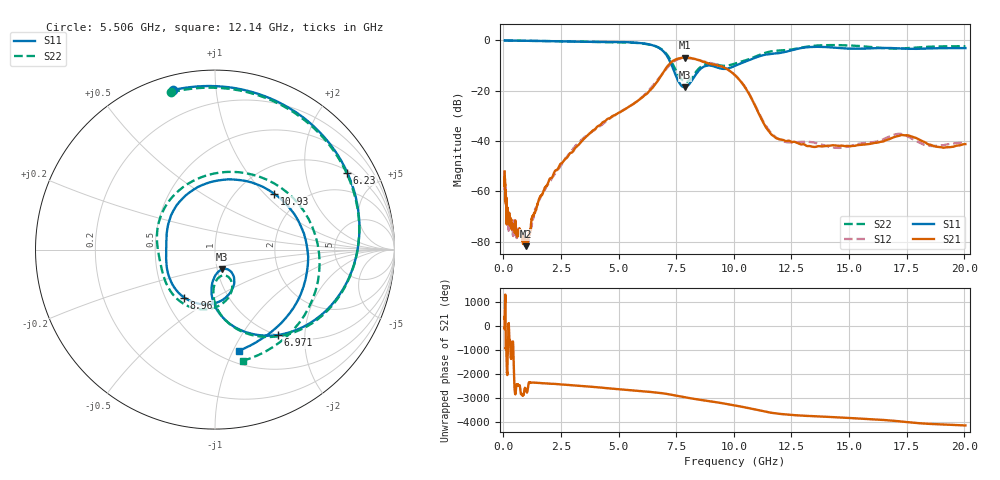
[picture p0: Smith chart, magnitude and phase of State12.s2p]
# Hz S DB R 50
!freq MagS11 AngS11 MagS21 AngS21 MagS12 AngS12 MagS22 AngS22
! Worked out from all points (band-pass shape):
!   1601 points, 50 MHz to 20.05 GHz, reference 50 ohm
!   highest |S21| = -6.81 dB at 7.859 GHz (marker M1); lowest = -81.9 dB at 964.4 MHz (marker M2)
!   |S21| within 3 dB of the highest: 7.16 GHz to 9.241 GHz (2.081 GHz wide, 25.4 % of centre)
!   lowest |S11| = -18.6 dB at 7.859 GHz (marker M3), VSWR 1.27, Z = 52.9 - j11.8 ohm
!   |S11| at or under -10 dB: 7.308 GHz to 8.859 GHz (1.551 GHz wide, 19.2 % of centre); 9.001 GHz to 10.07 GHz (1.069 GHz wide, 11.2 % of centre)
!   |S22| runs from -16.5 to 0.0 dB; largest |S21 - S12| = 0.024
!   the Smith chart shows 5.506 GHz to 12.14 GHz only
!   S11 on the Smith chart (normalised r, x): 5.506 GHz: 0.07, +0.77; 6.23 GHz: 1.08, +3.39; 6.971 GHz: 1.00, -1.46; 8.96 GHz: 0.62, -0.37; 10.93 GHz: 1.46, +1.14; 12.14 GHz: 0.62, -1.06
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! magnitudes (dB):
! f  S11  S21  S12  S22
! 50 MHz  0.0  -52.1  -51.8  0.0
! 72.18 MHz  0.0  -63.6  -60.0  0.0
! 135.9 MHz  0.0  -67.1  -65.3  0.0
! 144.3 MHz  0.0  -72.7  -66.7  0.0
! 174.7 MHz  0.0  -67.4  -71.3  0.0
! 208.4 MHz  0.0  -71.2  -69.6  0.0
! 226.3 MHz  0.0  -71.9  -75.2  0.0
! 369.6 MHz  0.0  -74.2  -75.1  0.0
! 517.8 MHz  -0.1  -71.6  -75.5  -0.1
! 964.4 MHz  -0.1  -81.9  -80.5  -0.1
! 1.005 GHz  -0.1  -80.0  -80.4  -0.1
! 2.722 GHz  -0.3  -46.9  -46.7  -0.4
! 5.506 GHz  -0.7  -26.0  -26.1  -0.8
! 6.23 GHz  -1.4  -21.2  -20.6  -1.4
! 6.971 GHz  -4.6  -12.3  -12.3  -4.3
! 7.402 GHz  -12.1  -7.9  -8.3  -10.4
! 7.859 GHz  -18.6  -6.8  -7.0  -16.4
! 8.96 GHz  -10.0  -9.2  -8.9  -9.1
! 10.03 GHz  -10.2  -13.6  -13.6  -9.2
! 10.93 GHz  -6.9  -26.1  -25.8  -6.4
! 12.14 GHz  -4.7  -39.6  -40.0  -3.9
! 20.05 GHz  -3.0  -41.2  -40.6  -2.3
